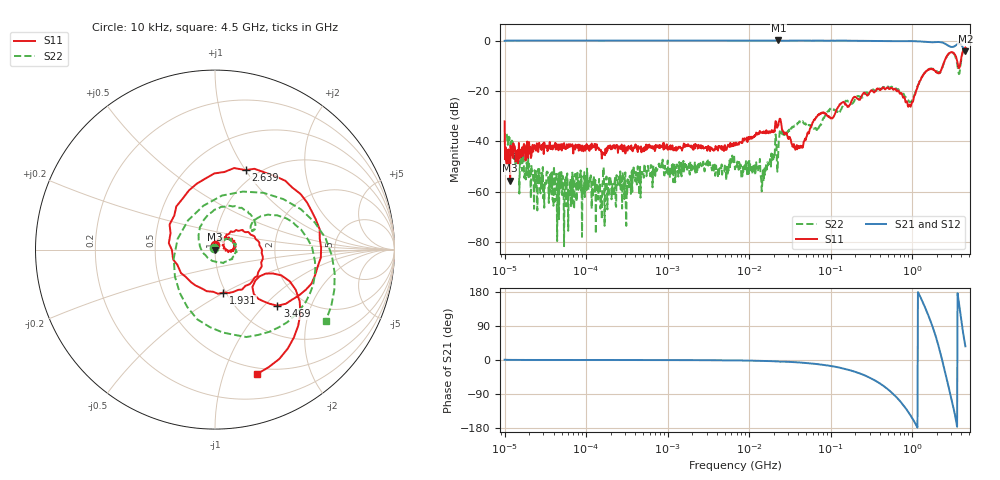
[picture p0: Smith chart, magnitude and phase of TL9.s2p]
!Siglent Technologies,SNA5004A,SNA5XCED5R0097,V1.0.0.2.10.R9
!Date: 2024-11-24 17:09:43
!Data & Calibration Information:
!Freq	S11:F2(ON)	S21:F2(ON)	S12:F2(ON)	S22:F2(ON)
# Hz S DB R 50
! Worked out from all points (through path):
!   1001 points, 10 kHz to 4.5 GHz, reference 50 ohm
!   highest |S21| = 0.11 dB at 22.8 MHz (marker M1); lowest = -4.2 dB at 4.5 GHz (marker M2)
!   group delay of S21, straight-line fit = 424 ps
!   lowest |S11| = -55.7 dB at 11.69 kHz (marker M3), VSWR 1.00, Z = 50.2 + j0.00308 ohm
!   |S11| at or under -10 dB: start of sweep to 2.371 GHz; 3.67 GHz to 3.855 GHz (185.9 MHz wide, 4.94 % of centre)
!   |S22| runs from -81.7 to -2.7 dB; largest |S21 - S12| = 0.021
!   S11 on the Smith chart (normalised r, x): 10 kHz: 1.00, +0.05; 1.931 GHz: 0.97, -0.50; 2.639 GHz: 0.88, +1.00; 3.469 GHz: 1.49, -1.20; 4.5 GHz: 0.43, -1.29
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10000  -32.11 89.9  -0.02 0.7  -0.03 0.8  -40.30 134.3
11690.65  -55.69 1.1  0.01 0.3  -0.04 0.2  -38.83 114.9
23920.22  -42.06 2.5  0.06 0.1  -0.01 -0.1  -58.88 165.3
87919.76  -43.84 5.8  0.06 0.0  -0.00 -0.1  -53.78 -76.8
772988.4  -42.33 15.3  0.07 -0.1  0.01 -0.3  -49.28 -46.5
6708204  -41.65 63.9  0.05 -1.1  -0.03 -1.3  -51.18 -136.5
1.484063e7  -36.76 97.0  0.05 -2.4  -0.03 -2.5  -51.47 -13.8
2.280385e7  -33.71 116.1  0.11 -3.8  0.03 -3.8  -43.85 100.2
3.939519e7  -41.78 121.6  0.06 -6.2  -0.04 -6.4  -32.68 83.6
5.897837e7  -33.53 56.4  0.02 -9.4  -0.05 -9.4  -34.05 96.4
2.313556e8  -23.17 52.1  -0.06 -36.0  -0.13 -35.8  -22.41 55.0
5.185364e8  -19.16 17.4  -0.15 -79.5  -0.21 -79.3  -18.50 3.1
8.072136e8  -22.56 -4.8  -0.17 -123.3  -0.22 -123.1  -22.05 -64.7
1.177421e9  -17.69 49.1  -0.23 179.3  -0.28 179.6  -17.88 134.3
1.588384e9  -11.38 -8.7  -0.57 116.6  -0.63 117.0  -11.43 61.9
1.930873e9  -12.26 -79.0  -0.55 65.0  -0.61 65.4  -11.73 30.0
2.286891e9  -11.55 159.6  -0.63 7.8  -0.70 8.3  -11.70 36.0
2.638948e9  -6.47 69.0  -1.53 -47.9  -1.56 -47.3  -6.57 16.9
3.045202e9  -4.63 5.9  -2.45 -103.6  -2.50 -102.8  -4.67 -29.9
3.468552e9  -6.60 -42.0  -1.73 -161.5  -1.79 -160.7  -7.25 -93.5
3.950758e9  -8.03 -21.2  -1.39 113.9  -1.45 115.2  -8.90 64.3
4.5e9  -2.70 -71.6  -4.24 36.1  -4.28 37.4  -2.68 -33.0
